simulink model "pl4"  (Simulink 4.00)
settings: Solver=ode45  StartTime=0.0  StopTime=8  RelTol=1e-3
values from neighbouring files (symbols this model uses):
  m = p    (= 10)    [scr1.m]    (also in scrmod1.m; scr.m; Smpc.m = mp(1:max(size(mp))-1); demo1dat.m = 4)
  model = tfd2step(tfinal,Ts,1,g)    [scr1.m]    (also in scrmod1.m = [y(2:ly); 1; 1; .1]; scr.m = [y(2:ly); 1; 1; .1]; Smpc.m = modelpd(:,1:nu); essai2dat.m = tfd2step(1.6,delt,1,g))
  p = 10    [scr1.m]    (also in scrmod1.m; scr.m; Smpc.m = mp(max(size(mp))); demo1dat.m)
  ulim = [-4 4 .5]    [scr1.m]    (also in scrmod1.m = []; scr.m; Smpc.m = [-inf*ones(1,nu) inf*ones(1,nu) 1e6*ones(1,nu)]; essai2dat.m = [-5 40 3])
  uwt = 1    [scr1.m]    (also in scrmod1.m; scr.m; Smpc.m = yuwt(:,ny+1:ny+nu); demo1dat.m = [0 0])
  ylim = [-inf inf]    [scr1.m]    (also in scrmod1.m = []; scr.m; Smpc.m = [ylim; ylim(N,:)]; essai2dat.m = [-40 40])
  ywt = 5    [scr1.m]    (also in scrmod1.m; scr.m; Smpc.m = yuwt(:,1:ny); demo1dat.m = [1 1])

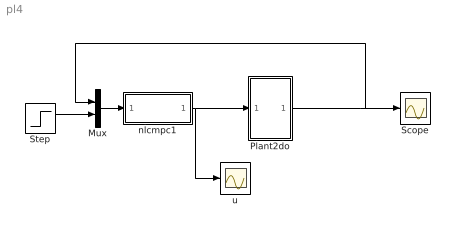
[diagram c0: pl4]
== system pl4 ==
  Mux : Mux  Inputs=2
  Plant2do : Subsystem
  Scope : Scope
  Step : Step  Time=1  Before=0  After=1  SampleTime=0
  nlcmpc1 : Subsystem  AncestorBlock=nlmpclib/nlcmpc  mask(Smpc){modelpd=[model []], yuwt=[ywt uwt], mp=[m p], yulim=[ylim ulim], tfilter=[], ud0=[0 []]}
      mask help: Masked MATLAB function block calls nlcmpc, links CMPC and SIMULINK.
  u : Scope
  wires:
  nlcmpc1/1(Out1) -> u/1, Plant2do/1(u)
  Mux/1 -> nlcmpc1/1(In1)
  Step/1 -> Mux/2
  Plant2do/1(y) -> Scope/1, Mux/1

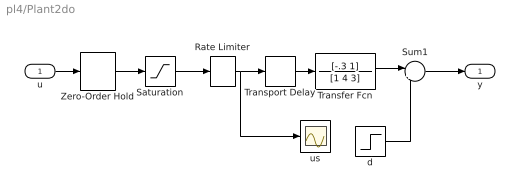
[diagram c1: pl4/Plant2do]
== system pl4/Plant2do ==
  u : Inport  Port=1  LatchInput=off
  Rate Limiter : RateLimiter  RisingSlewLimit=5  FallingSlewLimit=-5
  Saturation : Saturate  UpperLimit=4  LowerLimit=-4  LinearizeAsGain=on
  Sum1 : Sum  Inputs=|++  SaturateOnIntegerOverflow=on
  Transfer Fcn : TransferFcn  Numerator=[-.3 1]  Denominator=[1 4 3]  AbsoluteTolerance=auto  Realization=auto
  Transport Delay : TransportDelay  DelayTime=.2  InitialInput=0  BufferSize=1024  PadeOrder=0
  Zero-Order Hold : ZeroOrderHold  SampleTime=0.1
  d : Step  Time=4  Before=0  After=1  SampleTime=0
  us : Scope
  y : Outport  Port=1
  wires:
  Transport Delay/1 -> Transfer Fcn/1
  u/1 -> Zero-Order Hold/1
  Saturation/1 -> Rate Limiter/1
  Zero-Order Hold/1 -> Saturation/1
  Rate Limiter/1 -> Transport Delay/1, us/1
  d/1 -> Sum1/2
  Transfer Fcn/1 -> Sum1/1
  Sum1/1 -> y/1

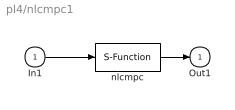
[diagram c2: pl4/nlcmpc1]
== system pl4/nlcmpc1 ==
  In1 : Inport  Port=1  LatchInput=off
  nlcmpc : S-Function  FunctionName=Smpc  Parameters=modelpd,mp,tfilter,yuwt,ud0,yulim  PortCounts=[]  SFunctionModules=''
  Out1 : Outport  Port=1  InitialOutput=0
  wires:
  In1/1 -> nlcmpc/1
  nlcmpc/1 -> Out1/1
